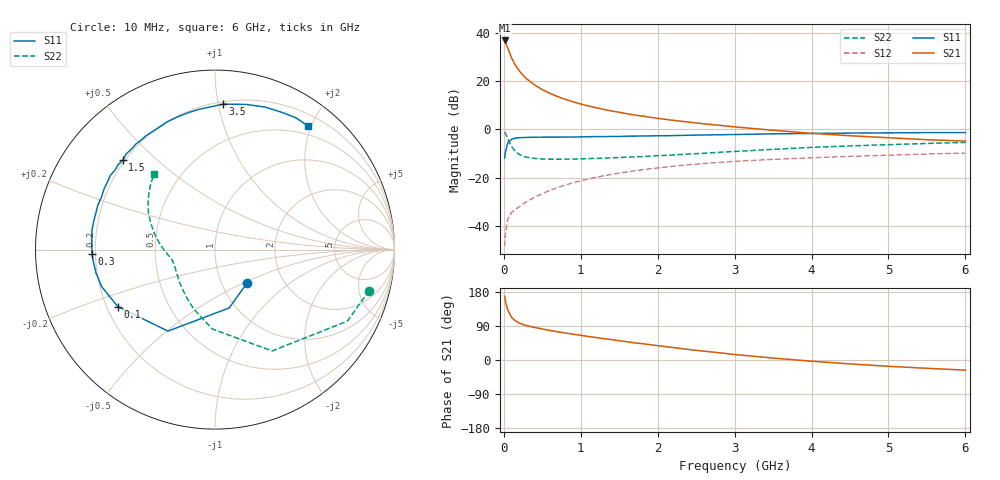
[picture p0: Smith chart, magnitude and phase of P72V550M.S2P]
! SIEMENS Small Signal Semiconductors
! BFP196
! Si NPN RF Bipolar Junction Transistor in SOT143
! VCE = 2.5 V  IC = 50 mA
! Common Emitter S-Parameters:  May  1996
# GHz  S  MA  R  50
!  f  S11  S21  S12  S22
! GHz  MAG  ANG  MAG  ANG  MAG  ANG  MAG  ANG
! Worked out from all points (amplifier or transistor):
!   36 points, 10 MHz to 6 GHz, reference 50 ohm
!   highest |S21| = 36.7 dB at 10 MHz (marker M1)
!   |S21| within 3 dB of that: start of sweep to 49.56 MHz
!   unconditionally stable (mu >= 1): 431.6 MHz to 4.198 GHz
!   at 250 MHz: K = 0.85, MSG = 26.5 dB, |S12| = -30.7 dB
!   at 1.4 GHz: K = 1.09, MAG = 11.3 dB, |S12| = -18.6 dB
!   at 6 GHz: K = 0.98, MSG = 2.5 dB, |S12| = -9.7 dB
!   S11 on the Smith chart (normalised r, x): 10 MHz: 1.32, -0.52; 100 MHz: 0.24, -0.26; 300 MHz: 0.19, -0.02; 1.5 GHz: 0.19, +0.39; 3.5 GHz: 0.22, +1.03; 6 GHz: 0.37, +1.96
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0.01  0.2578 -45.9  68.74 168.2  0.0039 80.3  0.8888 -14.9
0.02  0.3347 -76.4  64.26 156.3  0.0072 72.3  0.8383 -28.4
0.05  0.5243 -120.0  48.46 132.4  0.014 55.1  0.6481 -60.6
0.1  0.6276 -149.6  30.2 112.7  0.0194 48.6  0.4426 -92.0
0.15  0.664 -161.8  21.23 103.3  0.0225 49.2  0.3501 -110.0
0.2  0.6757 -168.9  16.31 97.5  0.0254 52.5  0.3059 -122.1
0.25  0.6813 -174.3  13.05 93.5  0.0292 54.5  0.2805 -131.4
0.3  0.686 -178.1  10.98 90.5  0.0324 57.0  0.2679 -137.6
0.4  0.6894 175.6  8.306 85.9  0.04 59.8  0.2523 -147.0
0.5  0.6938 171.4  6.647 81.9  0.0473 61.8  0.2456 -153.1
0.6  0.6943 166.9  5.549 78.0  0.0554 62.6  0.2435 -157.2
0.7  0.6943 162.7  4.772 74.3  0.0632 63.0  0.2434 -160.4
0.8  0.6981 159.4  4.177 71.3  0.0715 62.3  0.2441 -163.0
0.9  0.6968 155.3  3.715 68.1  0.0797 61.8  0.2447 -165.1
1.1  0.7073 148.3  3.057 62.0  0.095 60.3  0.2504 -168.4
1.5  0.7158 136.0  2.268 51.0  0.1257 55.4  0.2636 -173.7
2.2  0.7462 116.1  1.544 32.9  0.1744 45.3  0.2974 176.8
3  0.7864 96.6  1.131 14.5  0.2197 33.5  0.3514 164.7
3.5  0.8118 86.8  0.961 5.1  0.2415 26.6  0.389 157.3
4.5  0.8418 70.6  0.742 -10.3  0.2786 14.6  0.4575 144.6
5.5  0.8616 58.5  0.615 -21.9  0.3113 3.8  0.5143 134.0
6  0.8617 52.9  0.575 -26.8  0.326 -1.9  0.5399 128.8
